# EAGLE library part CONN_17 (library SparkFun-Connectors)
Multi connection point. Often used as Generic Header-pin footprint for 0.1 inch spaced/style header connections On any of the 0.1 inch spaced packages, you can populate with these: Break Away Headers - Straight (PRT-00116) Break Away Male Headers - Right Angle (PRT-00553) Female Headers (PRT-00115) Break Away Headers - Machine Pin (PRT-00117) Break Away Female Headers - Swiss Machine Pin (PRT-00743) For SCREWTERMINALS and SPRING TERMINALS visit here: Screw Terimnals on SparkFun.com (5mm/3.5mm/2.54mm spacing) This device is also useful as a general connection point to wire up your design to another part of your project. Our various solder wires solder well into these plated through hole pads. Hook-Up Wire - Assortment (Stranded, 22 AWG) (PRT-11375) Hook-Up Wire - Assortment (Solid Core, 22 AWG) (PRT-11367) View the entire wire category on our website here Special notes: Molex polarized connector foot print use with SKU : PRT-08231 with associated crimp pins and housings. 1MM SMD Version SKU: PRT-10208 NOTES ON THE VARIANTS LOCK and LOCK_LONGPADS... This footprint was designed to help hold the alignment of a through-hole component (i.e. 6-pin header) while soldering it into place. You may notice that each hole has been shifted either up or down by 0.005 of an inch from it's more standard position (which is a perfectly straight line). This slight alteration caused the pins (the squares in the middle) to touch the edges of the holes. Because they are alternating, it causes a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
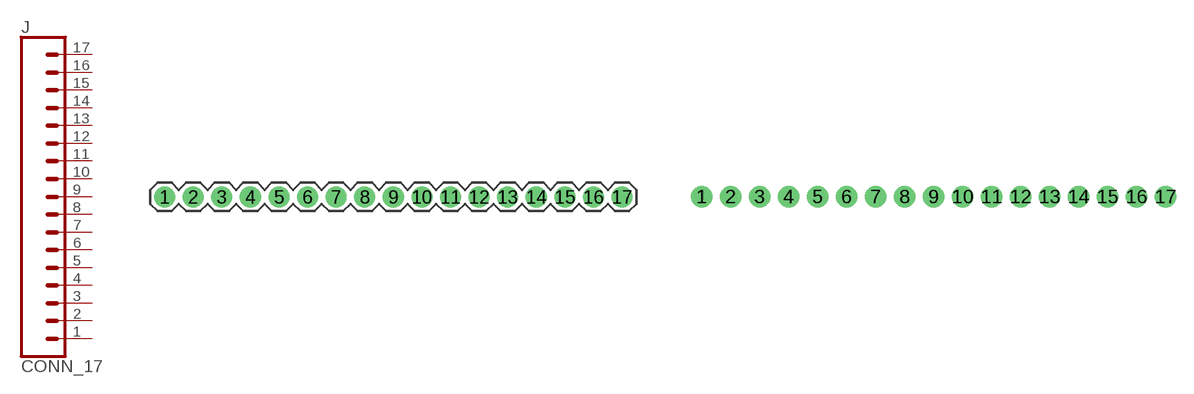
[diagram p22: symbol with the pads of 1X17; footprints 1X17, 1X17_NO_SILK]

Designator prefix J

## CONN_17  [1X17]
1  1  pas
2  2  pas
3  3  pas
4  4  pas
5  5  pas
6  6  pas
7  7  pas
8  8  pas
9  9  pas
10  10  pas
11  11  pas
12  12  pas
13  13  pas
14  14  pas
15  15  pas
16  16  pas
17  17  pas

## CONN_17NOSILK  [1X17_NO_SILK]
Pads as for 1X17

## CONN_17KIT (PROD_ID: CONN-12294)  [1X17_NO_SILK_KIT]
Pads as for 1X17

## Footprint 1X17 (pad centres in mm)
Plated Through Hole -17 Pin Specifications: Pin count:17 Pin pitch:0.1" Example device(s): CONN_17
drill 1.016 pad 1.88: 1 0,0; 2 2.54,0; 3 5.08,0; 4 7.62,0; 5 10.16,0; 6 12.7,0; 7 15.24,0; 8 17.78,0; 9 20.32,0; 10 22.86,0; 11 25.4,0; 12 27.94,0; 13 30.48,0; 14 33.02,0; 15 35.56,0; 16 38.1,0; 17 40.64,0

## Footprint 1X17_NO_SILK (pad centres in mm)
Plated Through Hole -17 Pin No Silk Specifications: Pin count:17 Pin pitch:0.1" Example device(s): CONN_17
drill 1.016 pad 1.88: 1 0,0; 2 2.54,0; 3 5.08,0; 4 7.62,0; 5 10.16,0; 6 12.7,0; 7 15.24,0; 8 17.78,0; 9 20.32,0; 10 22.86,0; 11 25.4,0; 12 27.94,0; 13 30.48,0; 14 33.02,0; 15 35.56,0; 16 38.1,0; 17 40.64,0

## Footprint 1X17_NO_SILK_KIT (pad centres in mm)
Plated Through Hole -17 Pin No Silk Kit Mask on only one side for soldering kits. Specifications: Pin count:17 Pin pitch:0.1" Example device(s): CONN_17
drill 1.016 pad 1.88: 1 0,0; 2 2.54,0; 3 5.08,0; 4 7.62,0; 5 10.16,0; 6 12.7,0; 7 15.24,0; 8 17.78,0; 9 20.32,0; 10 22.86,0; 11 25.4,0; 12 27.94,0; 13 30.48,0; 14 33.02,0; 15 35.56,0; 16 38.1,0; 17 40.64,0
